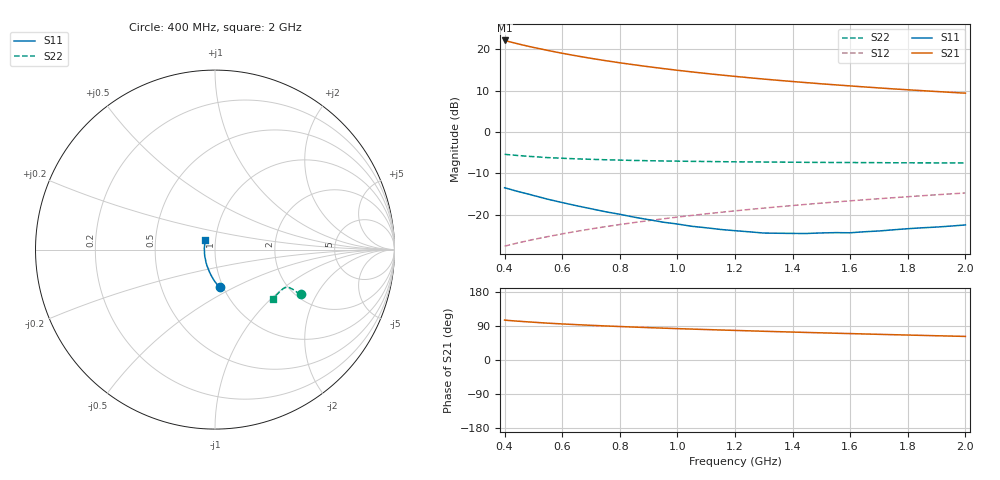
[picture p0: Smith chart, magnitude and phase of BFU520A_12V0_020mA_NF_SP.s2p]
! Filename:  P:\Prog\Test\Noise\ATS_data\Testdata_Net\06 Compressed Noise after Statistics\BFU520A_APG2013_30_A05_12p0V_020mA_NF_CM01_D.sf
! Date/Time: Wed 24/Apr/2013 20:06:22
! BFU520A_APG2013_30_A05_12p0V_1to20mA_NF_CM01_Bias8_R.sf
! Noise Parameter Data File
! BFU520A_APG2013_30_A05_12p0V_1to20mA_NF_CM01
! Date/time: Thu Apr 11 10:46:45 2013
! VAR V_out= 12.002000
! VAR I_out= 19.995000
! VAR V_in= 0.794900
! VAR I_in= 0.202300
! Device data file deembeded for feedlines and parallel
! Original file: \06 Compressed Noise after Statistics\BFU520A_APG2013_30_A05_12p0V_020mA_NF_CM01_R.sf
! Feed-files: PR017V01_150413_Feed1.s2p, PR017V01_150413_Feed2.s2p
! Parallel-file: PR017V01_150413_Par.s2p
# MHz S MA R 50
!  Freq-MHz  S11-mag  S11-arg  S21-mag  S21-arg  S12-mag  S12-arg  S22-mag  S22-arg
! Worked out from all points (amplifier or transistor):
!   37 points, 400 MHz to 2 GHz, reference 50 ohm
!   highest |S21| = 22.2 dB at 400 MHz (marker M1)
!   |S21| within 3 dB of that: start of sweep to 592.5 MHz
!   unconditionally stable (mu >= 1): 1.05 GHz to 1.957 GHz
!   at 500 MHz: K = 0.91, MSG = 23.2 dB, |S12| = -26.0 dB
!   at 1.1 GHz: K = 1.00, MAG = 16.8 dB, |S12| = -19.8 dB
!   at 2 GHz: K = 1.00, MSG = 12.1 dB, |S12| = -14.7 dB
!   lowest NFmin = 1.18 dB at 420 MHz
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400  0.2118 -83.1  12.85 105.2  0.04159 73.5  0.5382 -27.7
420  0.2026 -84.9  12.32 104.0  0.04332 73.6  0.5298 -27.6
440  0.1935 -86.7  11.84 102.8  0.04499 73.7  0.5226 -27.5
460  0.1857 -88.4  11.38 101.7  0.0467 73.9  0.5161 -27.5
500  0.171 -92.0  10.58 99.7  0.0501 74.1  0.5042 -27.3
550  0.1538 -96.1  9.736 97.2  0.05428 74.4  0.4909 -27.1
600  0.1403 -100.0  8.988 95.2  0.0586 74.6  0.4821 -27.0
650  0.1283 -103.8  8.357 93.3  0.06289 74.8  0.4741 -27.1
700  0.1181 -107.7  7.806 91.5  0.06724 74.9  0.4678 -27.1
750  0.1086 -111.6  7.321 89.9  0.07162 75.0  0.4623 -27.2
800  0.1012 -116.2  6.897 88.3  0.07599 75.0  0.4577 -27.4
850  0.09325 -120.5  6.519 86.8  0.08034 75.0  0.4534 -27.6
900  0.08714 -125.1  6.18 85.4  0.08472 74.9  0.4498 -27.9
950  0.08122 -129.4  5.874 84.1  0.08911 74.9  0.4471 -28.2
1050  0.0724 -138.8  5.347 81.6  0.09795 74.7  0.4421 -28.9
1150  0.06628 -150.1  4.911 79.2  0.1068 74.4  0.4382 -29.7
1200  0.06401 -155.1  4.721 78.1  0.1113 74.2  0.4366 -30.2
1350  0.05962 -171.5  4.229 74.7  0.1246 73.6  0.4329 -31.8
1500  0.06014 172.4  3.838 71.7  0.1381 72.9  0.4291 -33.5
1650  0.06217 159.2  3.518 68.7  0.1516 72.0  0.4272 -35.5
1750  0.06564 151.5  3.332 66.8  0.1605 71.4  0.425 -36.8
2000  0.07511 136.1  2.957 62.2  0.1832 69.9  0.4225 -40.5
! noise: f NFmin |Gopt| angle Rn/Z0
400  1.244  0.1585  -163.8  0.1109
460  1.19  0.1544  -161.7  0.1166
600  1.302  0.1472  -151.6  0.1299
800  1.265  0.181  -152.8  0.1104
1000  1.272  0.1936  -145.6  0.1148
1200  1.327  0.1961  -140  0.1228
1400  1.349  0.2127  -134.4  0.1234
1600  1.35  0.2344  -128.8  0.1269
1800  1.324  0.262  -127.8  0.1245
2000  1.349  0.2756  -123.3  0.1339
